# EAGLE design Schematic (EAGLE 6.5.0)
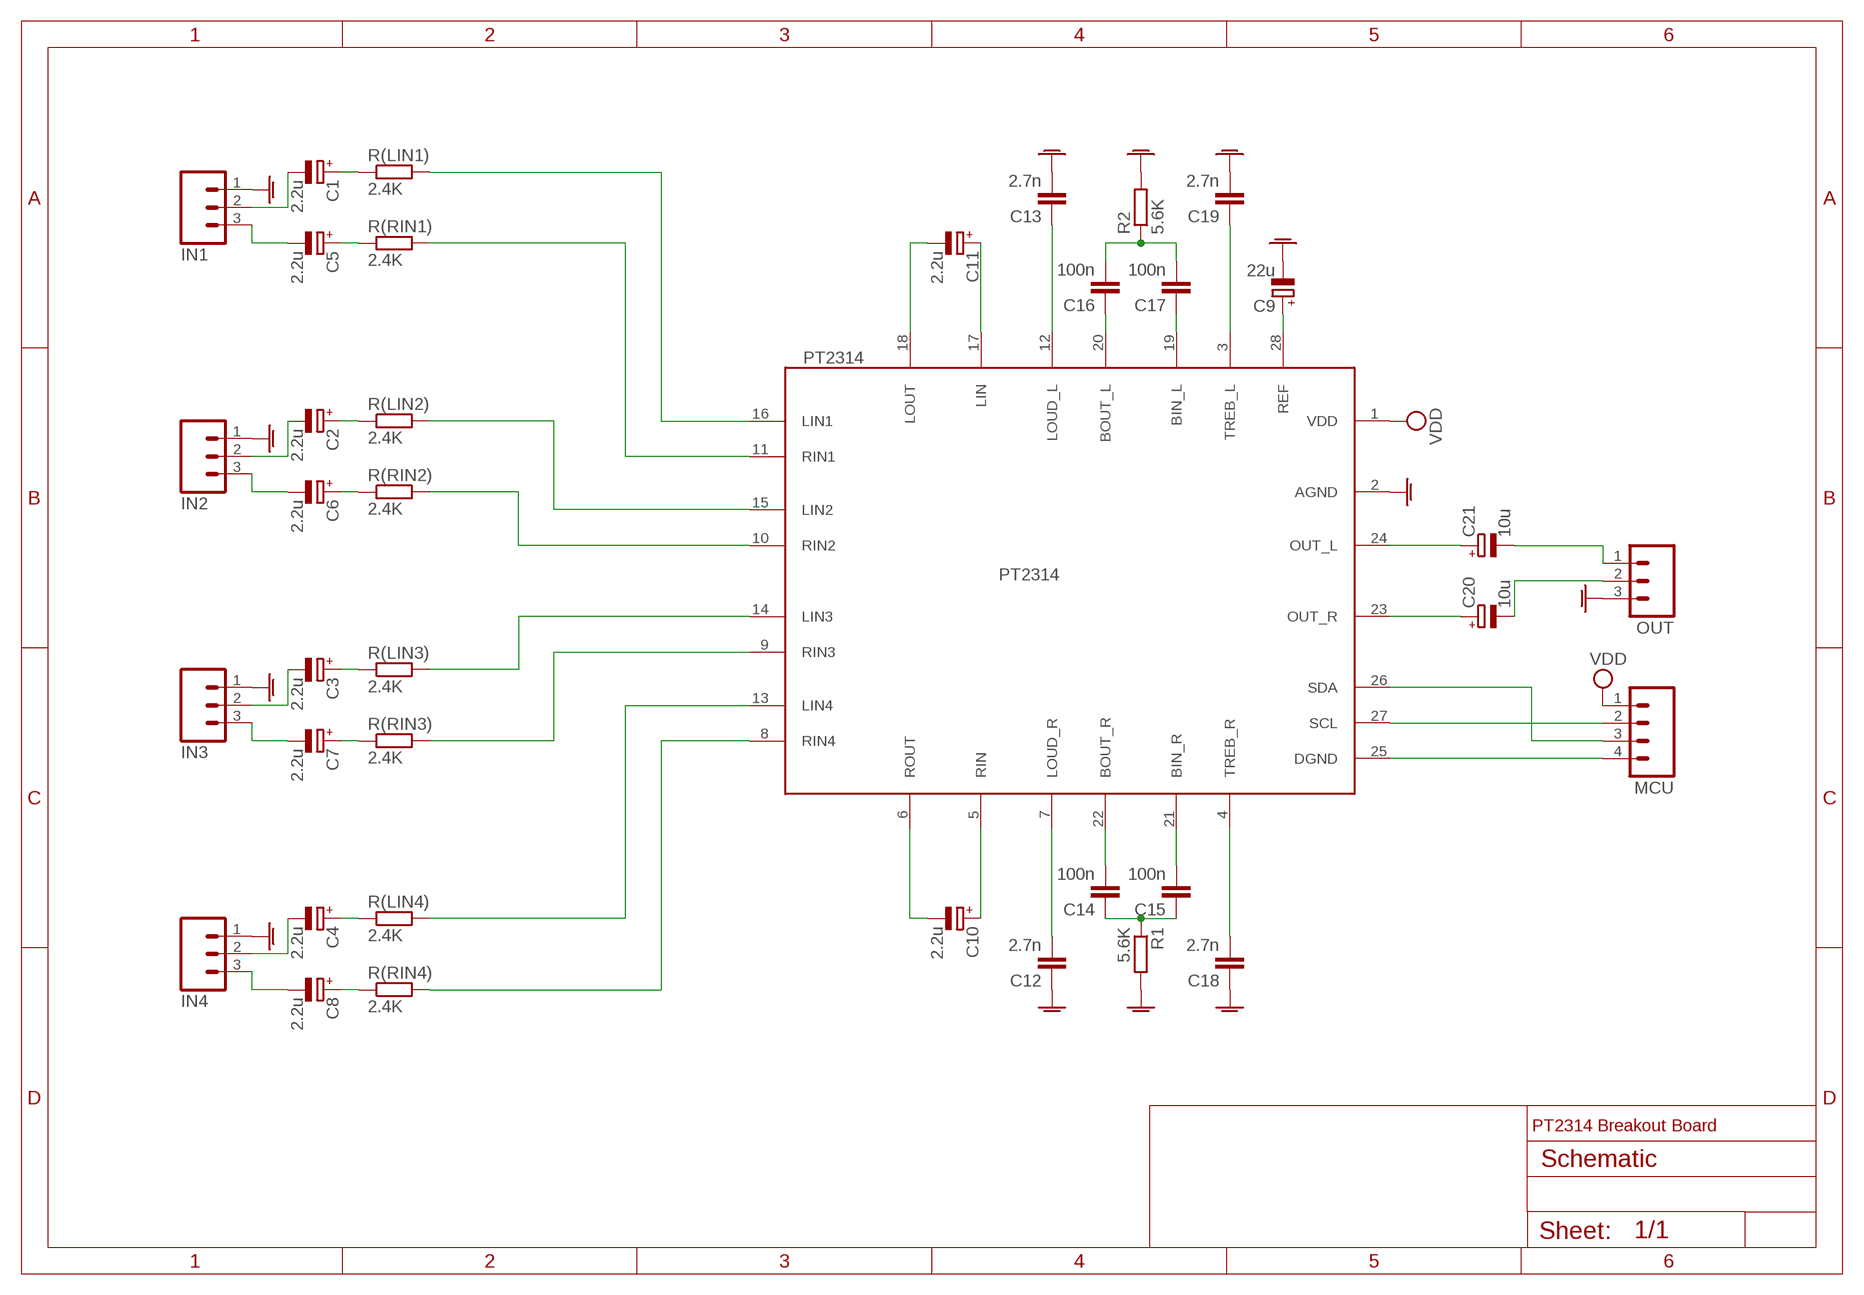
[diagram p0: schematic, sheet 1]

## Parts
C1  2.2u  CPOL-EUSMCZ  [SMC_Z]
C2  2.2u  CPOL-EUSMCZ  [SMC_Z]
C3  2.2u  CPOL-EUSMCZ  [SMC_Z]
C4  2.2u  CPOL-EUSMCZ  [SMC_Z]
C5  2.2u  CPOL-EUSMCZ  [SMC_Z]
C6  2.2u  CPOL-EUSMCZ  [SMC_Z]
C7  2.2u  CPOL-EUSMCZ  [SMC_Z]
C8  2.2u  CPOL-EUSMCZ  [SMC_Z]
C9  22u  CPOL-EUSMCZ  [SMC_Z]
C10  2.2u  CPOL-EUSMCZ  [SMC_Z]
C11  2.2u  CPOL-EUSMCZ  [SMC_Z]
C12  2.7n  C-EUC0603  [C0603]
C13  2.7n  C-EUC0603  [C0603]
C14  100n  C-EUC0603  [C0603]
C15  100n  C-EUC0603  [C0603]
C16  100n  C-EUC0603  [C0603]
C17  100n  C-EUC0603  [C0603]
C18  2.7n  C-EUC0603  [C0603]
C19  2.7n  C-EUC0603  [C0603]
C20  10u  CPOL-EUSMCZ  [SMC_Z]
C21  10u  CPOL-EUSMCZ  [SMC_Z]
IN1  M03PTH  [1X03]
IN2  M03PTH  [1X03]
IN3  M03PTH  [1X03]
IN4  M03PTH  [1X03]
MCU  M04PTH  [1X04]
OUT  M03PTH  [1X03]
PT2314  PT2314  [SO-28W]
R1  5.6K  R-EU_R0603  [R0603]
R2  5.6K  R-EU_R0603  [R0603]
R(LIN1)  2.4K  R-EU_R0603  [R0603]
R(LIN2)  2.4K  R-EU_R0603  [R0603]
R(LIN3)  2.4K  R-EU_R0603  [R0603]
R(LIN4)  2.4K  R-EU_R0603  [R0603]
R(RIN1)  2.4K  R-EU_R0603  [R0603]
R(RIN2)  2.4K  R-EU_R0603  [R0603]
R(RIN3)  2.4K  R-EU_R0603  [R0603]
R(RIN4)  2.4K  R-EU_R0603  [R0603]

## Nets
AGND: C9.- C12.1 C13.2 C18.1 C19.2 IN1.1 IN2.1 IN3.1 IN4.1 OUT.3 PT2314.2(AGND) R1.2 R2.2
B[IN|OUT]_L: C16.2 C17.2 R2.1
B[IN|OUT]_R: C14.1 C15.1 R1.1
BIN_L: C17.1 PT2314.19(BIN_L)
BIN_R: C15.2 PT2314.21(BIN_R)
BOUT_L: C16.1 PT2314.20(BOUT_L)
BOUT_R: C14.2 PT2314.22(BOUT_R)
C1-IN1_L: C1.- IN1.2
C1-R: C1.+ R(LIN1).1
C2-IN2_L: C2.- IN2.2
C2-R: C2.+ R(LIN2).1
C3-IN3_L: C3.- IN3.2
C3-R: C3.+ R(LIN3).1
C4-IN4_L: C4.- IN4.2
C4-R: C4.+ R(LIN4).1
C5-IN1_R: C5.- IN1.3
C5-R: C5.+ R(RIN1).1
C6-IN2_R: C6.- IN2.3
C6-R: C6.+ R(RIN2).1
C7-IN3_R: C7.- IN3.3
C7-R: C7.+ R(RIN3).1
C8-IN4_R: C8.- IN4.3
C8-R: C8.+ R(RIN4).1
C20-OUT_R: C20.- OUT.2
C21-OUT_L: C21.- OUT.1
DGND: MCU.4 PT2314.25(DGND)
LIN: C11.+ PT2314.17(LIN)
LIN1: PT2314.16(LIN1) R(LIN1).2
LIN2: PT2314.15(LIN2) R(LIN2).2
LIN3: PT2314.14(LIN3) R(LIN3).2
LIN4: PT2314.13(LIN4) R(LIN4).2
LOUT: C11.- PT2314.18(LOUT)
N$1: C19.1 PT2314.3(TREB_L)
N$2: C13.1 PT2314.12(LOUD_L)
N$3: C18.2 PT2314.4(TREB_R)
N$4: C12.2 PT2314.7(LOUD_R)
OUT_L: C21.+ PT2314.24(OUT_L)
OUT_R: C20.+ PT2314.23(OUT_R)
REF: C9.+ PT2314.28(REF)
RIN: C10.+ PT2314.5(RIN)
RIN1: PT2314.11(RIN1) R(RIN1).2
RIN2: PT2314.10(RIN2) R(RIN2).2
RIN3: PT2314.9(RIN3) R(RIN3).2
RIN4: PT2314.8(RIN4) R(RIN4).2
ROUT: C10.- PT2314.6(ROUT)
SCL: MCU.2 PT2314.27(SCL)
SDA: MCU.3 PT2314.26(SDA)
VDD: MCU.1 PT2314.1(VDD)

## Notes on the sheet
- PT2314 Breakout Board

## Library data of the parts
C1-C11 C20 C21 = rcl:CPOL-EU: POLARIZED CAPACITOR, European symbol
C12-C19 = rcl:C-EU: CAPACITOR, European symbol
IN1-IN4 OUT = SparkFun-Connectors:M03: Header 3 Standard 3-pin 0.1" header. Use with straight break away headers (SKU : PRT-00116), right angle break away headers (PRT-00553), swiss pins (PRT-00743), machine pins (PRT-00117), and female headers (PRT-00115). Molex polarized connector foot print use with SKU : PRT-08232 with associated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
MCU = SparkFun-Connectors:M04: Header 4 Standard 4-pin 0.1" header. Use with straight break away headers (SKU : PRT-00116), right angle break away headers (PRT-00553), swiss pins (PRT-00743), machine pins (PRT-00117), and female headers (PRT-00115). Molex polarized connector foot print use with SKU : PRT-08231 with associated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
PT2314 = audio-mixer-processor:PT2314: 4-Channel Input Audio Processor
R1 R2 R(LIN1) R(LIN2) R(LIN3) R(LIN4) R(RIN1) R(RIN2) R(RIN3) R(RIN4) = rcl:R-EU_: RESISTOR, European symbol

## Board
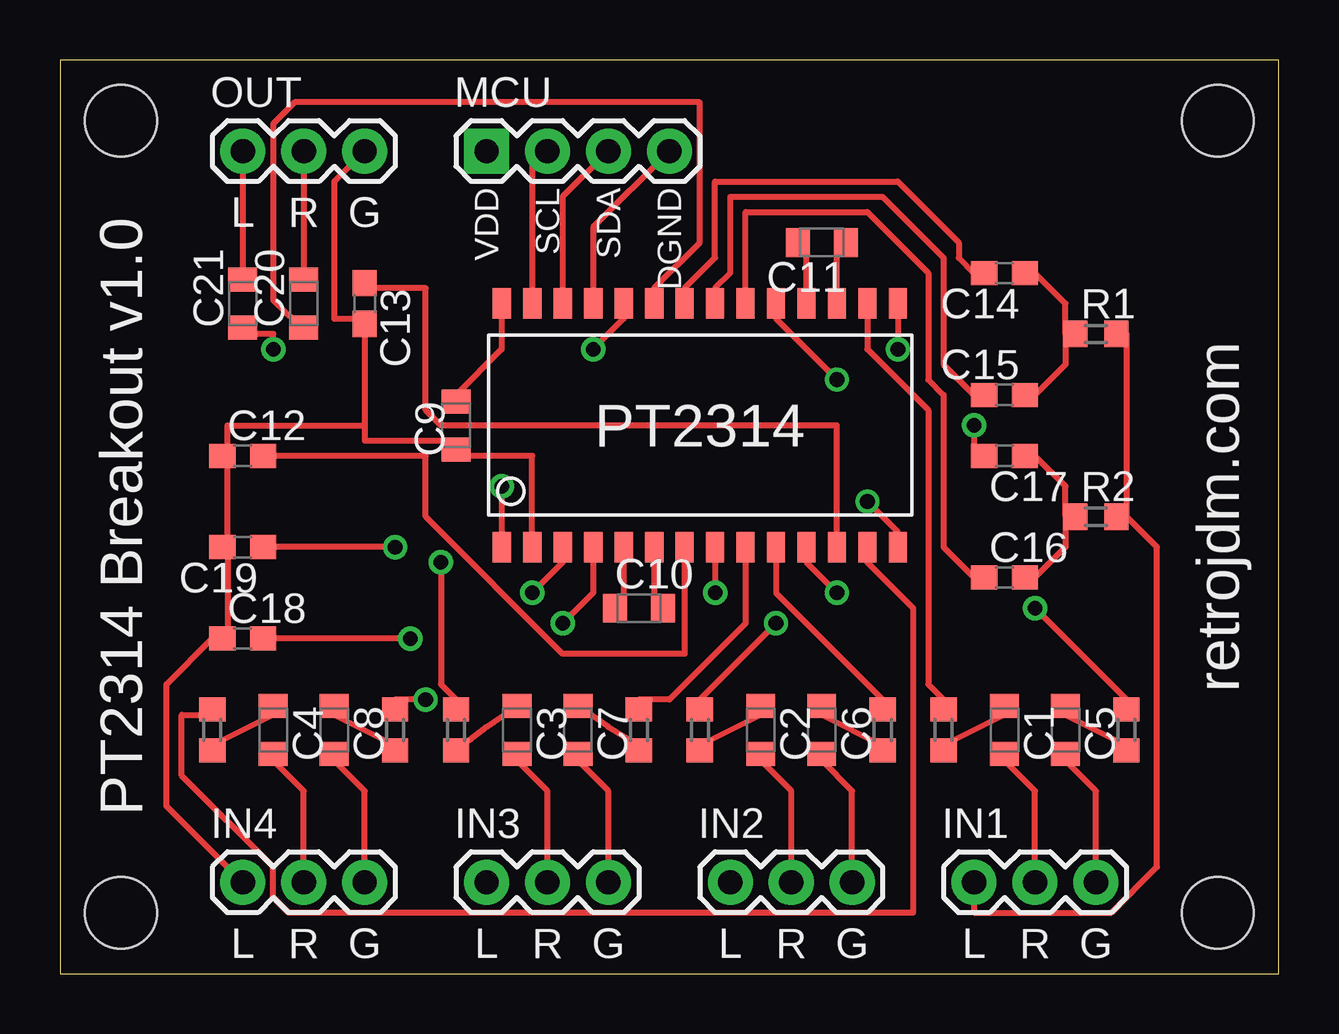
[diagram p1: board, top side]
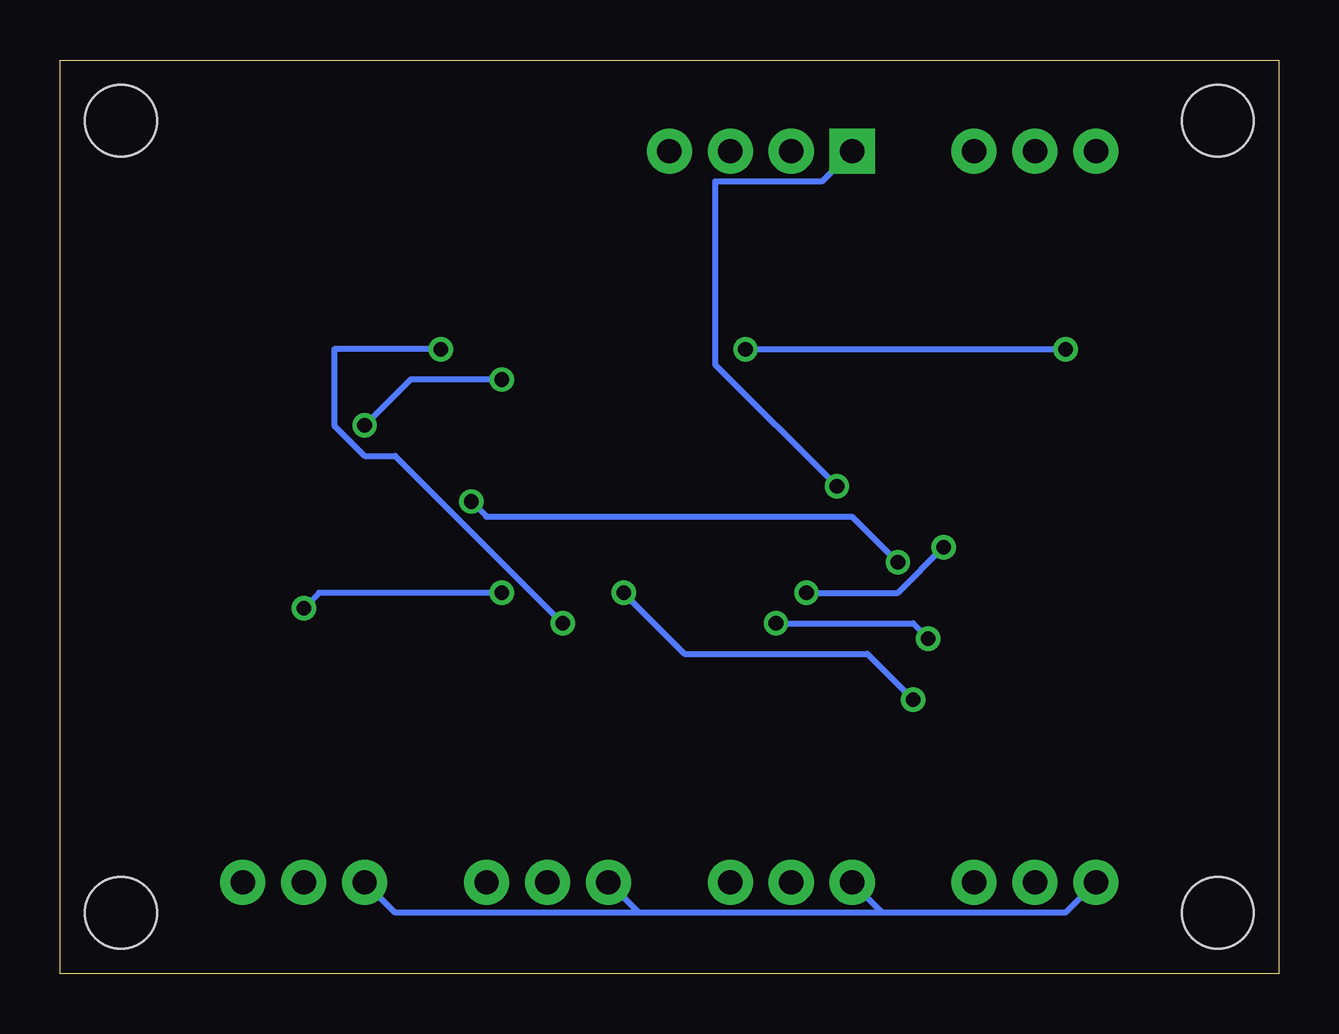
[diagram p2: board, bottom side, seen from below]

Size 50.8 x 38.09 mm. Coordinates in mm from the lower left corner, seen from the top.
Outline: 0,0 50.8,0 50.8,38.09 0,38.09 0,0
Copper layers (1*16): Top 0.035mm / dielectric 1.5mm / Bottom 0.035mm
Design rules "default": minimum track width 10mil, minimum drill 24mil, track to track 8mil, track to pad 8mil, pad to pad 8mil, via to via 8mil, smd to smd 8mil, copper to edge 40mil, drill to drill 8mil, minimum pad ring 10mil, minimum via ring 8mil, stop-mask expansion 4mil, vias tented up to drill 0mil, thermal gap 10mil
Holes 3 mm at 2.54,35.56 2.54,2.54 48.26,2.54 48.26,35.56

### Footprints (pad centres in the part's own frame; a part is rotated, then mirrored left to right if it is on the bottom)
SMC_Z = smd 1 x 1.2: + -1,0; - 1,0
C0603 = smd 1.1 x 1: 1 -0.85,0; 2 0.85,0
1X03 = drill 1.016 pad 1.88: 1 0,0; 2 2.54,0; 3 5.08,0
1X04 = drill 1.016 pad 1.88 square: 1 0,0 | drill 1.016 pad 1.88: 2 2.54,0; 3 5.08,0; 4 7.62,0
SO-28W = smd 0.762 x 1.27: 1 -8.255,-5.08; 2 -6.985,-5.08; 3 -5.715,-5.08; 4 -4.445,-5.08; 5 -3.175,-5.08; 6 -1.905,-5.08; 7 -0.635,-5.08; 8 0.635,-5.08; 9 1.905,-5.08; 10 3.175,-5.08; 11 4.445,-5.08; 12 5.715,-5.08; 13 6.985,-5.08; 14 8.255,-5.08; 15 8.255,5.08; 16 6.985,5.08; 17 5.715,5.08; 18 4.445,5.08; 19 3.175,5.08; 20 1.905,5.08; 21 0.635,5.08; 22 -0.635,5.08; 23 -1.905,5.08; 24 -3.175,5.08; 25 -4.445,5.08; 26 -5.715,5.08; 27 -6.985,5.08; 28 -8.255,5.08
R0603 = smd 1 x 1.1: 1 -0.85,0; 2 0.85,0

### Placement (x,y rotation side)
C1  39.37,10.16 270 top
C2  29.21,10.16 270 top
C3  19.05,10.16 270 top
C4  8.89,10.16 270 top
C5  41.91,10.16 270 top
C6  31.75,10.16 270 top
C7  21.59,10.16 270 top
C8  11.43,10.16 270 top
C9  16.51,22.86 270 top
C10  24.13,15.24 0 top
C11  31.75,30.48 180 top
C12  7.62,21.59 0 top
C13  12.7,27.94 270 top
C14  39.37,29.21 180 top
C15  39.37,24.13 180 top
C16  39.37,16.51 0 top
C17  39.37,21.59 0 top
C18  7.62,13.97 0 top
C19  7.62,17.78 180 top
C20  10.16,27.94 90 top
C21  7.62,27.94 90 top
IN1  38.1,3.81 0 top
IN2  27.94,3.81 0 top
IN3  17.78,3.81 0 top
IN4  7.62,3.81 0 top
MCU  17.78,34.29 0 top
OUT  7.62,34.29 0 top
PT2314  26.67,22.86 0 top
R1  43.18,26.67 0 top
R2  43.18,19.05 0 top
R(LIN1)  36.83,10.16 90 top
R(LIN2)  26.67,10.16 90 top
R(LIN3)  16.51,10.16 90 top
R(LIN4)  6.35,10.16 90 top
R(RIN1)  44.45,10.16 90 top
R(RIN2)  34.29,10.16 90 top
R(RIN3)  24.13,10.16 90 top
R(RIN4)  13.97,10.16 90 top

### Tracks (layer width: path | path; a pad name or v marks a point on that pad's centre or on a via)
AGND
  Top 0.254: 44.45,19.05 44.45,26.67 R1.2 | 44.45,19.05 45.72,17.78 45.72,4.45 43.81,2.54 38.1,2.54 IN1.1 | 44.45,19.05 R2.2 | PT2314.2 19.69,21.59 16.51,21.59 C9.- 16.51,22.23 12.7,22.23 12.7,22.86 | OUT.3 11.43,33.02 11.43,27.3 12.7,27.3 C13.2 12.7,22.86 | 6.99,17.78 6.99,13.97 C18.1 6.35,13.97 4.45,12.06 4.45,6.99 IN4.1 | 6.99,17.78 6.99,21.59 | 6.99,17.78 C19.2 | 12.7,22.86 6.99,22.86 6.99,21.59 | 6.99,21.59 C12.1
  Bottom 0.254: 16.51,2.54 IN3.1 | 16.51,2.54 8.89,2.54 IN4.1 | 26.67,2.54 IN2.1 | 16.51,2.54 26.67,2.54 | IN1.1 36.83,2.54 26.67,2.54
B[IN|OUT]_L
  Top 0.254: 41.91,19.05 41.91,17.78 40.64,16.51 C16.2 | 41.91,19.05 41.91,20.32 40.64,21.59 C17.2 | 41.91,19.05 R2.1
B[IN|OUT]_R
  Top 0.254: 41.91,26.67 41.91,25.4 40.64,24.13 C15.1 | 41.91,26.67 41.91,27.94 40.64,29.21 C14.1 | 41.91,26.67 R1.1
BIN_L  (via drill 0.61)
  Top 0.254: v38.1,22.86 38.1,21.59 C17.1 | v32.38,24.77 29.84,27.3 PT2314.19
  Bottom 0.254: v38.1,22.86 36.2,24.77 v32.38,24.77
BIN_R
  Top 0.254: PT2314.21 27.3,28.57 27.94,29.21 27.94,32.38 34.29,32.38 36.83,29.84 36.83,25.4 38.1,24.13 C15.2
BOUT_L
  Top 0.254: PT2314.20 28.58,31.75 33.66,31.75 36.2,29.21 36.2,24.77 36.83,24.13 36.83,17.78 38.1,16.51 C16.1
BOUT_R
  Top 0.254: PT2314.22 26.03,28.57 27.3,29.84 27.3,33.02 34.92,33.02 37.46,30.48 37.46,29.84 38.1,29.21 C14.2
C1-IN1_L
  Top 0.254: IN1.2 40.64,7.62 39.37,8.89 C1.-
C1-R
  Top 0.254: R(LIN1).1 36.83,9.53 39.37,10.79 C1.+
C2-IN2_L
  Top 0.254: IN2.2 30.48,7.62 29.21,8.89 C2.-
C2-R
  Top 0.254: R(LIN2).1 26.67,9.53 29.21,10.79 C2.+
C3-IN3_L
  Top 0.254: IN3.2 20.32,7.62 19.05,8.89 C3.-
C3-R
  Top 0.254: R(LIN3).1 17.78,10.29 C3.+
C4-IN4_L
  Top 0.254: IN4.2 10.16,7.62 8.89,8.89 C4.-
C4-R
  Top 0.254: R(LIN4).1 6.35,9.53 8.89,10.79 C4.+
C5-IN1_R
  Top 0.254: IN1.3 43.18,7.62 41.91,8.89 C5.-
C5-R
  Top 0.254: R(RIN1).1 44.45,9.53 41.91,10.79 C5.+
C6-IN2_R
  Top 0.254: IN2.3 33.02,7.62 31.75,8.89 C6.-
C6-R
  Top 0.254: R(RIN2).1 34.29,9.53 31.75,10.79 C6.+
C7-IN3_R
  Top 0.254: IN3.3 22.86,7.62 21.59,8.89 C7.-
C7-R
  Top 0.254: R(RIN3).1 24.13,9.53 22.86,10.29 C7.+
C8-IN4_R
  Top 0.254: IN4.3 12.7,7.62 11.43,8.89 C8.-
C8-R
  Top 0.254: R(RIN4).1 13.97,9.53 11.43,10.79 C8.+
C20-OUT_R
  Top 0.254: OUT.2 C20.-
C21-OUT_L
  Top 0.254: OUT.1 C21.-
DGND
  Top 0.254: PT2314.25 22.23,31.11 MCU.4
LIN
  Top 0.254: PT2314.17 32.38,30.48 C11.+
LIN1
  Top 0.254: PT2314.16 33.66,26.04 36.2,23.5 36.2,12.06 36.83,11.43 R(LIN1).2
LIN2  (via drill 0.61)
  Top 0.254: v29.84,14.61 26.67,11.43 R(LIN2).2 | PT2314.15 v34.92,26.04
  Bottom 0.254: v29.84,14.61 36.83,21.59 38.1,21.59 39.37,22.86 39.37,26.04 v34.92,26.04
LIN3  (via drill 0.61)
  Top 0.254: v15.88,17.14 15.88,12.06 16.51,11.43 R(LIN3).2 | v33.66,19.68 34.92,18.41 PT2314.14
  Bottom 0.254: v15.88,17.14 17.78,19.05 33.02,19.05 v33.66,19.68
LIN4
  Top 0.254: PT2314.13 33.66,17.14 35.56,15.24 35.56,2.54 9.53,2.54 8.89,3.17 8.89,4.45 5.08,8.26 5.08,10.79 6.35,10.79 R(LIN4).2
LOUT
  Top 0.254: PT2314.18 31.12,30.48 C11.-
N$1  (via drill 0.61)
  Top 0.254: v13.97,17.78 C19.1 | v19.69,15.88 20.95,17.14 PT2314.3
  Bottom 0.254: v13.97,17.78 15.88,15.88 v19.69,15.88
N$2
  Top 0.254: PT2314.12 32.38,22.86 15.88,22.86 15.24,23.5 15.24,28.57 12.7,28.57 C13.1
N$3  (via drill 0.61)
  Top 0.254: v14.61,13.97 C18.2 | v20.95,14.61 22.23,15.88 PT2314.4
  Bottom 0.254: v14.61,13.97 15.24,14.61 v20.95,14.61
N$4
  Top 0.254: C12.2 15.24,21.59 15.24,19.05 20.95,13.34 26.03,13.34 PT2314.7
OUT_L  (via drill 0.61)
  Top 0.254: v8.89,26.04 8.89,26.67 7.62,26.67 C21.+ | v22.23,26.04 23.49,27.3 PT2314.24
  Bottom 0.254: v22.23,26.04 v8.89,26.04
OUT_R
  Top 0.254: PT2314.23 24.77,28.57 26.67,30.48 26.67,36.32 9.78,36.32 8.89,35.43 8.89,28.07 9.4,27.56 C20.+
REF
  Top 0.254: PT2314.28 18.41,26.04 16.51,24.13 C9.+
RIN
  Top 0.254: PT2314.5 23.49,15.24 C10.+
RIN1  (via drill 0.61)
  Top 0.254: v40.64,15.24 44.45,11.43 R(RIN1).2 | v32.38,15.88 31.12,17.14 PT2314.11
  Bottom 0.254: v40.64,15.24 40,15.88 v32.38,15.88
RIN2
  Top 0.254: PT2314.10 29.84,15.88 34.29,11.43 R(RIN2).2
RIN3
  Top 0.254: PT2314.9 28.58,14.61 25.4,11.43 24.13,11.43 R(RIN3).2
RIN4  (via drill 0.61)
  Top 0.254: v15.24,11.43 13.97,11.43 R(RIN4).2 | PT2314.8 v27.3,15.88
  Bottom 0.254: v15.24,11.43 17.14,13.34 24.77,13.34 v27.3,15.88
ROUT
  Top 0.254: PT2314.6 24.77,15.24 C10.-
SCL
  Top 0.254: PT2314.27 19.69,33.66 MCU.2
SDA
  Top 0.254: PT2314.26 20.95,32.38 MCU.3
VDD  (via drill 0.61)
  Top 0.254: v18.41,20.32 PT2314.1
  Bottom 0.254: v18.41,20.32 23.49,25.4 23.49,33.02 19.05,33.02 MCU.1

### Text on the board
tNames: VDD | SCL | SDA | DGND | L | R | G | PT2314 Breakout v1.0 | retrojdm.com | L | R | G | L | R | G | L | R | G | L | R | G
